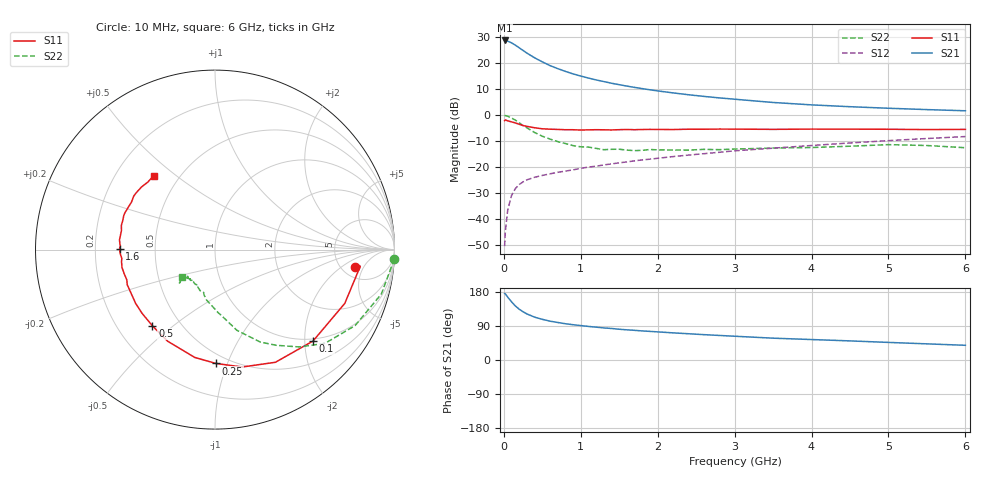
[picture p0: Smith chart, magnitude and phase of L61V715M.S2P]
!  INFINEON TECHNOLOGIES Small Signal Semiconductors
! BFR380L3 , Si-NPN RF-Transistor in TSLP-3-1
!  Vce=1.75 V,  Ic=15 mA
! Common Emitter S-Parameters:  07. March 2005
#  GHz  S  MA  R  50
! f  S11  S21  S12  S22
! GHz  Mag  Ang  Mag  Ang  Mag  Ang  Mag  Ang
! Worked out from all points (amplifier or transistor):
!   36 points, 10 MHz to 6 GHz, reference 50 ohm
!   highest |S21| = 28.9 dB at 10 MHz (marker M1)
!   |S21| within 3 dB of that: start of sweep to 207.7 MHz
!   unconditionally stable (mu >= 1): 1.982 GHz to 4.874 GHz
!   at 250 MHz: K = 0.32, MSG = 25.3 dB, |S12| = -25.7 dB
!   at 1.4 GHz: K = 0.93, MSG = 15.6 dB, |S12| = -18.8 dB
!   at 6 GHz: K = 0.98, MSG = 5.0 dB, |S12| = -8.2 dB
!   S11 on the Smith chart (normalised r, x): 10 MHz: 6.67, -3.36; 100 MHz: 0.95, -2.19; 250 MHz: 0.43, -0.91; 500 MHz: 0.35, -0.42; 1.6 GHz: 0.31, +0.00; 6 GHz: 0.36, +0.42
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0.01  0.787 -7.0  27.71 175.4  0.003 81.8  0.9999 -3.0
0.02  0.8149 -6.5  27.59 174.5  0.0059 87.0  0.9848 -6.2
0.05  0.7828 -22.5  26.89 166.0  0.0148 80.4  0.9597 -14.9
0.1  0.7469 -43.0  24.89 153.5  0.0285 69.7  0.888 -28.5
0.15  0.7123 -61.8  22.49 142.6  0.0386 62.4  0.8049 -40.5
0.2  0.6715 -76.9  19.97 134.0  0.0463 58.2  0.7176 -49.1
0.25  0.6346 -89.4  17.77 127.3  0.052 53.5  0.6328 -57.4
0.3  0.6114 -100.6  15.79 121.5  0.057 52.0  0.5736 -63.9
0.4  0.5746 -117.4  12.84 113.1  0.0638 48.8  0.4661 -74.8
0.5  0.5494 -129.4  10.71 107.3  0.0693 48.3  0.3951 -81.2
0.6  0.5395 -139.0  9.096 102.5  0.0744 48.6  0.3481 -87.7
0.7  0.5341 -145.9  7.938 99.0  0.0796 49.3  0.311 -93.6
0.9  0.5267 -158.2  6.277 93.1  0.0887 51.2  0.2603 -103.5
1.1  0.5237 -165.3  5.216 88.6  0.1005 53.3  0.2438 -109.7
1.4  0.5214 -174.6  4.148 83.2  0.1154 56.0  0.2211 -117.3
1.6  0.5318 179.6  3.653 79.6  0.1262 56.7  0.2131 -125.3
2.2  0.5317 168.7  2.702 71.6  0.16 59.4  0.214 -129.8
2.8  0.5428 159.3  2.166 64.8  0.1935 60.7  0.2175 -136.7
3.5  0.5354 150.3  1.767 57.6  0.2325 59.9  0.2338 -136.7
4.5  0.5406 143.5  1.464 50.4  0.2931 59.5  0.2536 -137.1
5.5  0.5306 134.9  1.287 42.6  0.3567 56.6  0.2615 -137.5
6  0.5354 129.7  1.222 38.8  0.3891 54.8  0.237 -140.0
